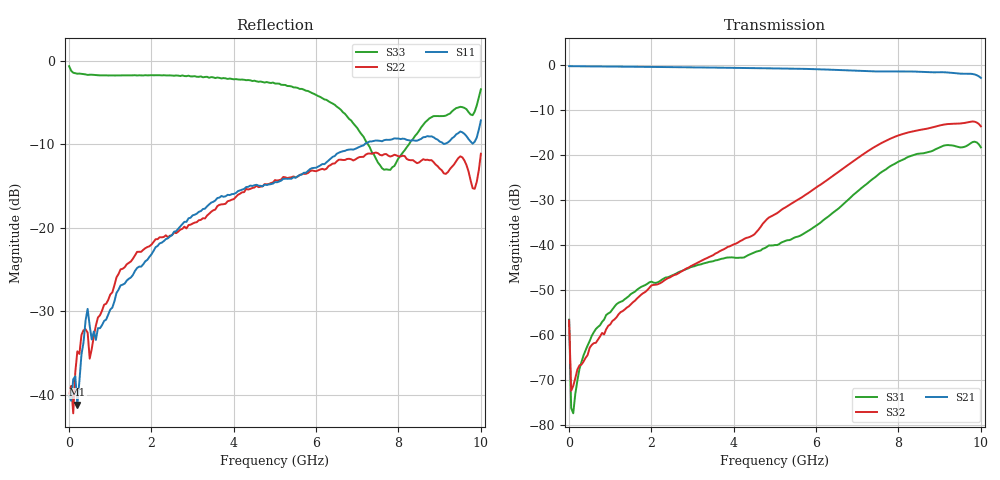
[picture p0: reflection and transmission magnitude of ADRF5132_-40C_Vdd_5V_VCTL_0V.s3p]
! Device:  ADRF5132
! Description: Silicon SPDT Switch
! Frequency:  0.7 -  5 GHz
! Ports:
!	RFc	= Port 1
!	RF1	= Port 2
!  RF2  = Port 3
! Vdd:  5 Volt
! Control:  0/0 Volt
! Data:  Data was collected using a calibrated 4 port network analyzer and de-embedded using AtaiTec's In Situ De-Embedding.
! Note:  Analog Devices supplies this data as a sample of measured data
!  for this product.  Your particular data for this product may vary.
!  Data was taken at -40 degrees C.
!  Analog Devices reserves the right to change this data at anytime.
# GHZ S DB R 50.0
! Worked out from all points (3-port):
!   201 points, 10 MHz to 10 GHz, reference 50 ohm
!   strongest paths, dB at 10 MHz, 2.507 GHz, 5.005 GHz, 7.503 GHz, 10 GHz:
!     S21: -0.3, -0.5, -0.8, -1.5, -2.9
!     S32: -56.8, -46.9, -33.2, -17.8, -13.7
!     S31: -56.6, -46.8, -40.0, -24.5, -18.4
!   lowest |S11| = -41.2 dB at 209.8 MHz (marker M1), VSWR 1.02, Z = 50.4 - j0.754 ohm
!   |S11| at or under -10 dB: start of sweep to 7.176 GHz
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0.01  -40.16 44.7  -0.33 -0.3  -57.30 -58.5
      -0.34 -0.3  -39.86 40.9  -57.34 -55.8
      -56.60 -59.4  -56.77 -61.5  -0.62 -8.3
0.05995  -40.73 -22.1  -0.35 -1.1  -73.93 -43.0
         -0.36 -1.1  -38.94 -13.4  -71.72 -42.5
         -76.23 -54.2  -72.39 -38.1  -1.17 -41.9
0.2098  -41.19 -58.9  -0.34 -3.7  -70.31 67.9
        -0.36 -3.7  -34.80 -27.5  -68.66 -30.2
        -70.17 67.5  -67.68 -31.9  -1.52 -105.2
0.45955  -29.71 -94.4  -0.38 -8.1  -62.33 79.6
         -0.39 -8.1  -32.56 -90.6  -64.54 -62.9
         -62.32 77.5  -64.44 -62.4  -1.67 -146.9
1.15885  -27.81 -116.3  -0.43 -19.9  -53.18 81.3
         -0.44 -19.8  -25.94 -90.4  -56.00 -108.8
         -53.17 80.9  -56.08 -108.5  -1.73 -179.7
5.005  -14.52 144.7  -0.82 -84.9  -40.03 -7.1
       -0.84 -84.6  -14.28 -147.2  -33.19 -179.1
       -40.03 -6.8  -33.21 -179.4  -2.70 108.7
7.65235  -9.49 99.4  -1.49 -130.7  -23.42 -177.7
         -1.51 -130.2  -11.18 171.0  -17.07 107.8
         -23.49 -177.0  -17.10 107.5  -13.03 87.0
8.9011  -9.32 74.8  -1.68 -153.8  -18.75 109.3
        -1.70 -153.3  -12.41 154.3  -13.73 54.0
        -18.77 109.8  -13.74 53.6  -6.60 107.0
9.65035  -9.00 62.1  -2.00 -167.3  -18.02 74.6
         -2.03 -166.6  -12.47 137.8  -12.84 27.6
         -18.06 74.9  -12.86 27.0  -5.78 88.6
10  -7.12 25.3  -2.91 172.2  -18.29 21.3
    -2.94 172.9  -11.11 88.3  -13.66 -0.6
    -18.35 21.5  -13.69 -1.2  -3.39 18.6
